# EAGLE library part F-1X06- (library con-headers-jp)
FEMALE HEADER
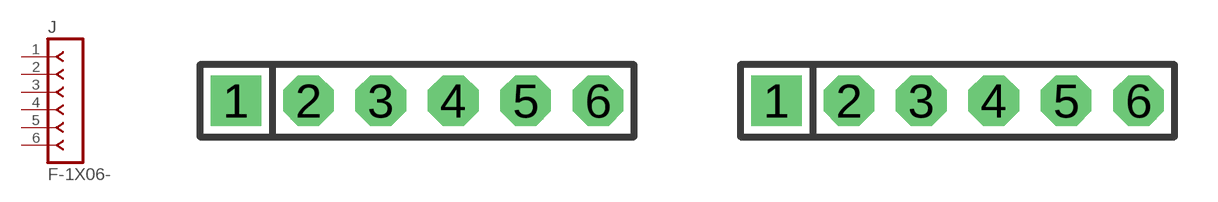
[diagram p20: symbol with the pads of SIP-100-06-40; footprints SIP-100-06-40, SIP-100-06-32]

Designator prefix J

## F-1X06-SIP-100-40  [SIP-100-06-40]
1  1  pas
2  2  pas
3  3  pas
4  4  pas
5  5  pas
6  6  pas

## F-1X06-SIP-100-32  [SIP-100-06-32]
Pads as for SIP-100-06-40

## F-1X06-SIP-100-32Y  [SIP-100-06-32Y]
Pads as for SIP-100-06-40

## F-1X06-SIP-100-40Y  [SIP-100-06-40Y]
Pads as for SIP-100-06-40

## F-1X06-KK-4455-B06  [KK-4455-B06]
Pads as for SIP-100-06-40

## F-1X06-KK-4455-C06  [KK-4455-C06]
Pads as for SIP-100-06-40

## F-1X06-KK-4455-A06  [KK-4455-A06]
Pads as for SIP-100-06-40

## Footprint SIP-100-06-40 (pad centres in mm)
SIP Header - 0.1", 40 mil drill
drill 1.016 pad 1.778 square: 1 -6.35,0
drill 1.016 pad 1.778 octagon: 2 -3.81,0; 3 -1.27,0; 4 1.27,0; 5 3.81,0; 6 6.35,0

## Footprint SIP-100-06-32 (pad centres in mm)
SIP Header - 0.1", 32 mil drill
drill 0.813 pad 1.778 square: 1 -6.35,0
drill 0.813 pad 1.778 octagon: 2 -3.81,0; 3 -1.27,0; 4 1.27,0; 5 3.81,0; 6 6.35,0

## Footprint SIP-100-06-32Y (pad centres in mm)
SIP Header - 0.1", 32 mil drill
drill 0.813 long: 1 -6.35,0; 2 -3.81,0; 3 -1.27,0; 4 1.27,0; 5 3.81,0; 6 6.35,0

## Footprint SIP-100-06-40Y (pad centres in mm)
SIP Header - 0.1", 40 mil drill
drill 1.016 long: 1 -6.35,0; 2 -3.81,0; 3 -1.27,0; 4 1.27,0; 5 3.81,0; 6 6.35,0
